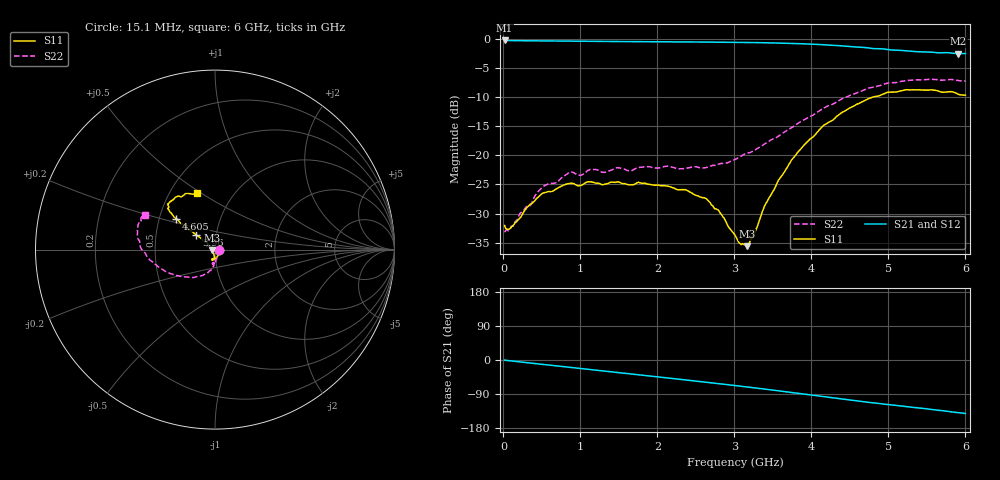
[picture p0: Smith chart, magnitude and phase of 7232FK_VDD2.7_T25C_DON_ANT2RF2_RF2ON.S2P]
!Agilent Technologies,E5071C,MY46417908,A.11.23
!Date: Fri Mar 03 11:28:32 2017
!Data & Calibration Information:
!Freq	S11:SOLT2(ON)	S21:SOLT2(ON)	S12:SOLT2(ON)	S22:SOLT2(ON)
!PortZ  Port1:50+j0  Port2:50+j0
!Above PortZ is port z conversion or system Z0 setting when saving the data.
!When reading, reference impedance value at option line is always used.
# Hz S dB R 50
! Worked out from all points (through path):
!   400 points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, 15.1 MHz to 6 GHz, reference 50 ohm
!   highest |S21| = -0.26 dB at 15.1 MHz (marker M1); lowest = -2.5 dB at 5.91 GHz (marker M2)
!   group delay of S21, straight-line fit = 65.8 ps
!   lowest |S11| = -35.6 dB at 3.165 GHz (marker M3), VSWR 1.03, Z = 48.4 - j0.385 ohm
!   |S11| at or under -10 dB: start of sweep to 4.796 GHz
!   |S22| runs from -33.2 to -6.9 dB; largest |S21 - S12| = 0.0068
!   S11 on the Smith chart (normalised r, x): 15.1 MHz: 1.05, -0.01; 3.96 GHz: 0.80, +0.14; 4.605 GHz: 0.61, +0.23; 6 GHz: 0.68, +0.48
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1.509975e7  -32.06 -9.1  -0.26 -0.4  -0.25 -0.5  -33.24 -9.0
7.509875e7  -32.68 -25.6  -0.28 -1.8  -0.28 -1.8  -32.89 -26.8
5.250912e8  -26.44 -83.6  -0.35 -11.9  -0.35 -11.9  -25.29 -81.2
8.550858e8  -24.83 -99.2  -0.39 -19.2  -0.39 -19.2  -22.92 -88.2
1.020083e9  -25.09 -101.8  -0.40 -22.8  -0.40 -22.8  -23.35 -89.9
1.140081e9  -24.56 -104.3  -0.42 -25.5  -0.42 -25.5  -22.40 -92.0
2.010066e9  -25.12 -103.4  -0.49 -44.6  -0.48 -44.6  -22.20 -100.2
2.640056e9  -27.50 -95.0  -0.54 -58.9  -0.54 -58.9  -22.06 -96.2
2.790054e9  -29.38 -100.5  -0.56 -62.4  -0.56 -62.4  -21.51 -96.4
3.01505e9  -33.92 -117.9  -0.59 -67.6  -0.58 -67.6  -20.69 -95.6
3.075049e9  -35.21 -135.2  -0.59 -69.0  -0.59 -69.0  -20.20 -96.2
3.165047e9  -35.61 -166.1  -0.62 -71.2  -0.61 -71.2  -19.65 -97.8
3.390044e9  -28.74 152.3  -0.66 -76.7  -0.65 -76.7  -18.06 -105.2
3.57004e9  -24.33 142.3  -0.71 -81.3  -0.70 -81.2  -16.72 -111.7
3.960034e9  -17.49 141.4  -0.88 -91.4  -0.88 -91.4  -13.51 -133.1
4.005033e9  -17.00 142.2  -0.90 -92.6  -0.89 -92.5  -13.21 -135.7
4.17003e9  -14.75 142.5  -1.02 -97.1  -1.01 -97.0  -11.81 -145.8
4.605023e9  -11.16 141.5  -1.40 -108.1  -1.40 -108.1  -9.19 -167.0
5.010016e9  -9.14 139.0  -1.85 -117.9  -1.84 -117.8  -7.55 176.6
5.490008e9  -8.79 130.5  -2.22 -128.8  -2.22 -128.7  -6.97 163.7
5.910002e9  -9.51 112.4  -2.53 -138.9  -2.52 -138.8  -7.16 154.4
6e9  -9.67 107.8  -2.50 -141.2  -2.53 -141.0  -7.23 153.6
